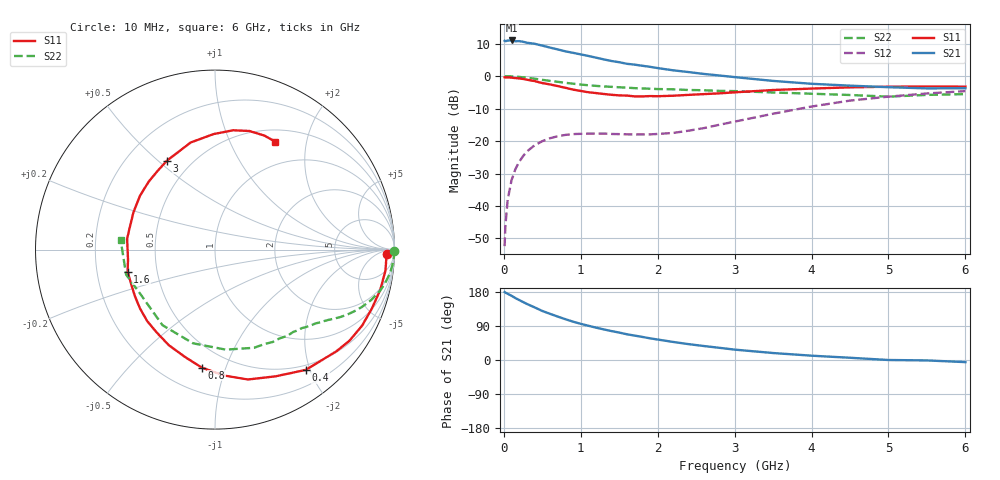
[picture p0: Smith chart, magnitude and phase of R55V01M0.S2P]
! SIEMENS Small Signal Semiconductors
! BFR183
! Si NPN RF Bipolar Junction Transistor in SOT23
! VCE = 5 V  IC = 1 mA
! Common Emitter S-Parameters:  May  1996
# GHz  S  MA  R  50
!  f  S11  S21  S12  S22
! GHz  MAG  ANG  MAG  ANG  MAG  ANG  MAG  ANG
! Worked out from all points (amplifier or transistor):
!   36 points, 10 MHz to 6 GHz, reference 50 ohm
!   highest |S21| = 11.0 dB at 100 MHz (marker M1)
!   |S21| within 3 dB of that: start of sweep to 740.8 MHz
!   unconditionally stable (mu >= 1): 1.663 GHz to 2.947 GHz
!   at 250 MHz: K = 0.15, MSG = 17.6 dB, |S12| = -24.6 dB
!   at 1.4 GHz: K = 0.85, MSG = 11.2 dB, |S12| = -17.8 dB
!   at 6 GHz: K = 0.95, MSG = 0.4 dB, |S12| = -4.6 dB
!   S11 on the Smith chart (normalised r, x): 10 MHz: 36, -22; 400 MHz: 0.43, -1.93; 800 MHz: 0.35, -0.83; 1.6 GHz: 0.34, -0.11; 3 GHz: 0.37, +0.53; 6 GHz: 0.66, +1.50
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0.01  0.9601 -1.4  3.515 179.3  0.0024 93.1  0.9983 -0.4
0.02  0.9558 -2.7  3.451 177.8  0.0049 84.8  0.9929 -0.9
0.05  0.957 -7.0  3.533 174.7  0.0125 85.3  0.9976 -2.5
0.1  0.9476 -13.7  3.55 169.5  0.0249 82.7  0.9919 -5.0
0.15  0.9336 -20.6  3.452 163.4  0.0369 77.4  0.9845 -7.5
0.2  0.9227 -27.3  3.465 158.2  0.048 73.5  0.9732 -9.8
0.25  0.9051 -34.1  3.391 153.0  0.0586 69.6  0.9599 -12.1
0.4  0.8394 -53.0  3.157 138.9  0.086 59.5  0.9143 -17.9
0.5  0.7824 -64.5  2.954 129.4  0.0996 53.5  0.878 -21.4
0.6  0.7465 -75.8  2.756 121.9  0.1105 48.3  0.8463 -24.1
0.8  0.662 -96.3  2.414 107.7  0.1244 40.1  0.79 -28.5
0.9  0.6204 -105.8  2.289 101.1  0.128 37.5  0.7653 -30.2
1.1  0.5648 -125.0  2.047 90.3  0.1302 33.5  0.7237 -33.5
1.3  0.5313 -141.8  1.812 80.7  0.1306 31.3  0.6946 -36.3
1.6  0.502 -165.9  1.551 67.9  0.127 31.8  0.6654 -40.5
1.9  0.4932 173.1  1.393 57.2  0.1267 37.9  0.6398 -45.1
2.2  0.4995 155.5  1.231 47.7  0.1333 44.6  0.627 -50.0
3  0.5631 118.4  0.967 27.4  0.1992 57.7  0.5888 -68.3
3.5  0.612 102.8  0.845 18.4  0.2637 56.7  0.5604 -83.9
4.5  0.6725 81.4  0.714 5.9  0.4203 43.7  0.5127 -124.8
5.5  0.6923 66.6  0.648 -1.1  0.5414 26.7  0.5144 -164.3
6  0.6887 60.7  0.652 -5.6  0.5882 16.6  0.5285 174.1
